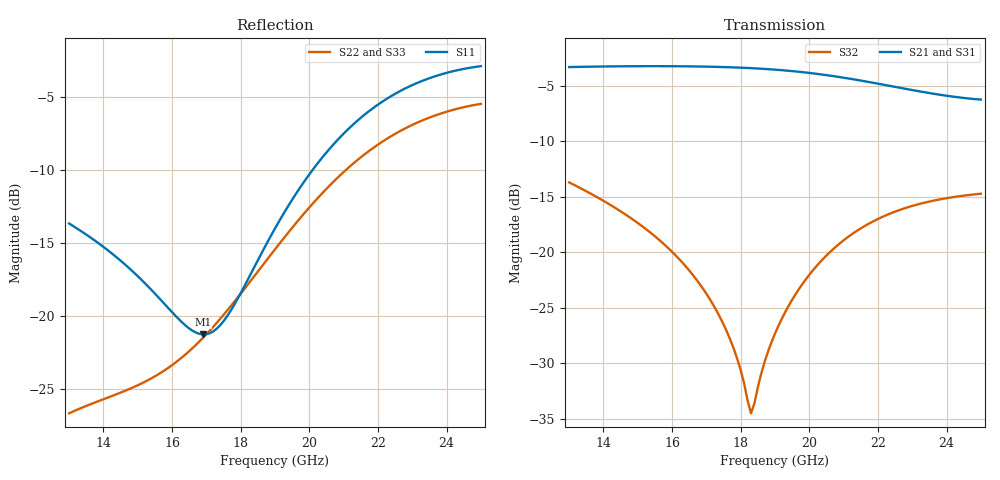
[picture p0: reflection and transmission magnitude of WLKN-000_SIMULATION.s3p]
! Generated from HFSS CSV (module + angle)
! Frequency range 13.000 to 25.000 GHz
# GHZ S RI R 50.0
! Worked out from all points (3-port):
!   121 points, 13 GHz to 25 GHz, reference 50 ohm
!   strongest paths, dB at 13 GHz, 16 GHz, 19 GHz, 22 GHz, 25 GHz:
!     S21: -3.3, -3.2, -3.5, -4.8, -6.2
!     S31: -3.3, -3.2, -3.5, -4.8, -6.2
!     S32: -13.7, -20.0, -27.3, -17.0, -14.7
!   lowest |S11| = -21.3 dB at 16.9 GHz (marker M1), VSWR 1.19, Z = 42.1 - j1.3 ohm
!   |S11| at or under -10 dB: start of sweep to 20.09 GHz
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13  0.1723 -0.1156  -0.3394 0.5934  -0.3392 0.5931
    -0.3394 0.5934  0.0166 -0.0435  0.0588 0.1979
    -0.3392 0.5931  0.0588 0.1979  0.0296 -0.0363
14.9  0.0162 -0.1396  0.1103 0.6808  0.1102 0.6805
      0.1103 0.6808  0.0261 0.051  0.1101 0.0848
      0.1102 0.6805  0.1101 0.0848  0.0267 0.0511
16.9  -0.0852 -0.0154  0.5375 0.4281  0.5372 0.428
      0.5375 0.4281  -0.0472 0.0698  0.0683 0.00522
      0.5372 0.428  0.0683 0.00522  -0.0472 0.0707
17.7  -0.081 0.0652  0.6359 0.2468  0.6356 0.2468
      0.6359 0.2468  -0.0303 0.1035  0.0402 -0.002
      0.6356 0.2468  0.0402 -0.002  -0.0302 0.1044
18.3  -0.0522 0.1298  0.6693 0.0948  0.669 0.0948
      0.6693 0.0948  -0.00739 0.1323  0.0187 0.00157
      0.669 0.0948  0.0187 0.00157  -0.00726 0.1332
19  0.0141 0.199  0.66 -0.086  0.6597 -0.0858
    0.66 -0.086  0.0349 0.1656  0.00741 0.0423
    0.6597 -0.0858  0.00741 0.0423  0.0351 0.1666
20.4  0.2431 0.2541  0.4947 -0.393  0.4945 -0.3927
      0.4946 -0.393  0.176 0.1983  0.0461 0.0811
      0.4945 -0.3927  0.0461 0.0811  0.1763 0.1995
21.7  0.4811 0.1312  0.2338 -0.5382  0.2338 -0.5378
      0.2338 -0.5382  0.3382 0.1358  0.1125 0.0721
      0.2338 -0.5378  0.1125 0.0721  0.3387 0.1373
23.3  0.6068 -0.1999  -0.0792 -0.5225  -0.079 -0.5221
      -0.0792 -0.5225  0.4633 -0.0644  0.1662 -0.00961
      -0.079 -0.5222  0.1662 -0.00961  0.4642 -0.0626
25  0.4675 -0.5434  -0.3104 -0.3765  -0.31 -0.3764
    -0.3104 -0.3765  0.434 -0.3086  0.1406 -0.118
    -0.31 -0.3764  0.1406 -0.118  0.4355 -0.3067
